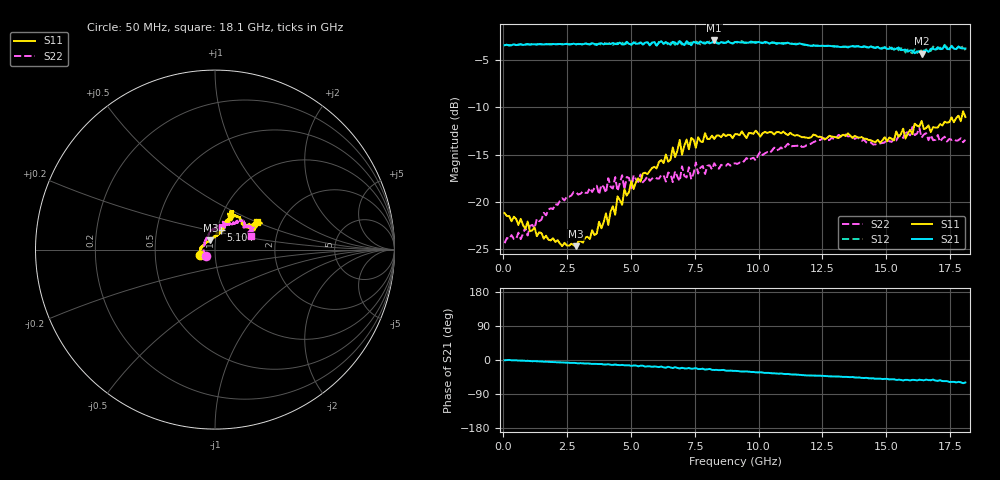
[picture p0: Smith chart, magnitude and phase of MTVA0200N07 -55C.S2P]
! Network Analyzer HP8720D.06.14 Serial No. US36140669
! 21 Jun 2005  11:45:47
! Frequency  S11  S21  S12  S22
# HZ  S  DB R 50
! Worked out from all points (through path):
!   201 points, 50 MHz to 18.1 GHz, reference 50 ohm
!   highest |S21| = -2.95 dB at 8.263 GHz (marker M1); lowest = -4.4 dB at 16.39 GHz (marker M2)
!   group delay of S21, straight-line fit = 9.45 ps
!   lowest |S11| = -24.7 dB at 2.848 GHz (marker M3), VSWR 1.12, Z = 47.2 + j4.98 ohm
!   |S11| at or under -10 dB: start of sweep to end of sweep
!   |S22| runs from -24.3 to -12.1 dB; largest |S21 - S12| = 0.037
!   S11 on the Smith chart (normalised r, x): 50 MHz: 0.85, -0.05; 5.104 GHz: 1.04, +0.24; 18.1 GHz: 1.51, +0.51
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5e7  -21.16 -160.0  -3.45 -0.6  -3.46 -0.3  -24.34 -144.6
2.84775e9  -24.66 116.1  -3.36 -8.3  -3.36 -8.2  -18.97 97.2
3.1185e9  -24.28 109.5  -3.36 -8.7  -3.41 -9.1  -18.87 97.5
4.021e9  -21.20 86.0  -3.28 -11.9  -3.33 -11.1  -19.03 86.7
4.11125e9  -22.41 83.5  -3.30 -11.1  -3.33 -12.6  -17.48 86.0
5.01375e9  -17.81 72.7  -3.38 -15.6  -3.43 -14.6  -18.57 79.3
5.104e9  -18.63 72.8  -3.15 -14.5  -3.21 -15.6  -17.17 78.4
6.09675e9  -15.76 65.5  -3.19 -18.7  -3.10 -18.5  -17.54 75.7
6.7285e9  -15.26 69.6  -3.18 -18.8  -3.43 -19.9  -16.75 69.2
6.909e9  -13.45 66.8  -3.01 -22.4  -3.12 -20.8  -17.81 69.1
6.99925e9  -15.01 66.1  -3.25 -20.6  -3.38 -22.7  -16.23 69.5
7.36025e9  -13.24 59.4  -3.46 -23.1  -3.16 -22.2  -17.60 74.6
7.54075e9  -14.26 61.5  -3.19 -21.4  -3.06 -24.2  -15.82 74.5
7.90175e9  -12.73 64.6  -3.30 -25.2  -3.18 -23.8  -17.04 69.0
8.26275e9  -13.35 66.4  -2.95 -26.3  -3.16 -27.1  -15.90 63.3
9.075e9  -12.83 66.6  -3.13 -28.8  -3.10 -29.0  -15.91 63.0
1.21435e10  -12.89 64.0  -3.49 -40.7  -3.45 -41.1  -13.69 51.9
1.512175e10  -13.20 37.4  -3.83 -51.3  -3.64 -51.3  -13.59 37.2
1.602425e10  -12.84 34.4  -4.02 -52.3  -4.29 -54.9  -12.09 29.6
1.638525e10  -11.44 29.0  -4.36 -52.7  -4.01 -52.1  -13.21 28.1
1.674625e10  -12.62 30.4  -3.83 -53.3  -4.07 -54.4  -12.94 24.9
1.81e10  -11.03 33.4  -3.80 -59.4  -3.98 -59.9  -13.44 21.5
